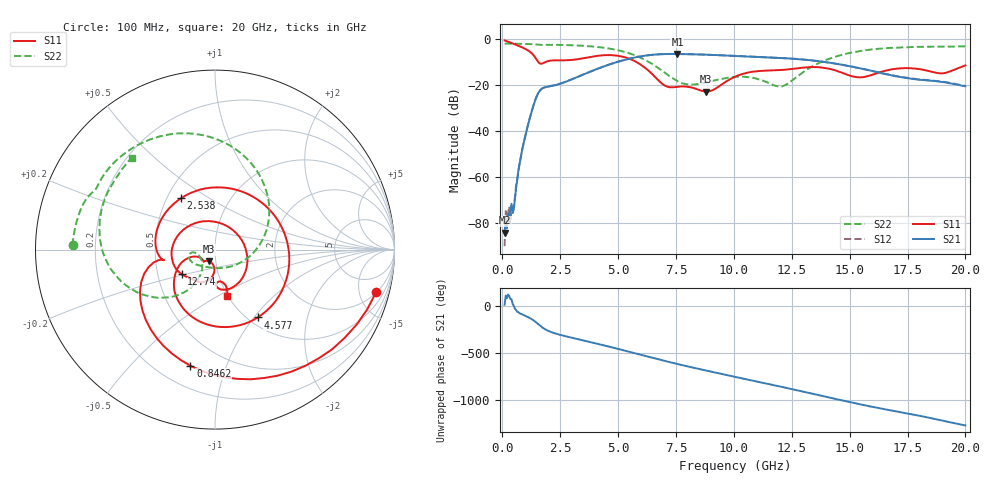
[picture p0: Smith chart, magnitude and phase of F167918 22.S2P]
!  2-Port S-parameters saved by WinCal
! VAR MeasName=S-Parameters (CALIBRATED_DATA) read from VNA (N5242A)
! VAR MeasDate=2016-11-22 10:25:49
! VAR NAME=F167918 22
! VAR FILENAME=F167918 22.S2P
! VAR DATE=2016-11-22 10:25:49
! VAR PHYS_PORTS=1,2
# Hz S DB R 50
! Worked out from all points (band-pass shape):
!   401 points, 100 MHz to 20 GHz, reference 50 ohm
!   highest |S21| = -6.49 dB at 7.562 GHz (marker M1); lowest = -84.2 dB at 100 MHz (marker M2)
!   |S21| within 3 dB of the highest: 5.137 GHz to 13.52 GHz (8.382 GHz wide, 89.9 % of centre)
!   lowest |S11| = -22.8 dB at 8.806 GHz (marker M3), VSWR 1.16, Z = 46.5 - j6.02 ohm
!   |S11| at or under -10 dB: 1.556 GHz to 1.868 GHz (311.8 MHz wide, 18.2 % of centre); 5.793 GHz to end of sweep
!   |S22| runs from -20.7 to -2.0 dB; largest |S21 - S12| = 0.005
!   S11 on the Smith chart (normalised r, x): 100 MHz: 2.07, -7.12; 846.2 MHz: 0.33, -0.76; 2.538 GHz: 0.59, +0.38; 4.577 GHz: 1.11, -1.04; 12.74 GHz: 0.66, -0.19; 20 GHz: 0.99, -0.55
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1e8  -0.64 -14.8  -84.16 17.5  -89.97 57.8  -2.00 178.3
4.4825e8  -1.91 -57.8  -75.62 26.3  -72.96 21.5  -2.05 172.6
8.4625e8  -3.59 -101.9  -48.76 -83.0  -48.78 -82.8  -2.11 166.1
1.1945e9  -5.56 -140.1  -34.13 -126.2  -34.08 -126.1  -2.21 160.2
1.54275e9  -9.85 -169.4  -23.71 171.9  -23.66 171.8  -2.48 154.7
2.53775e9  -9.29 123.3  -19.32 52.4  -19.29 52.1  -2.58 139.5
3.43325e9  -8.50 36.7  -15.71 -0.8  -15.72 -0.9  -2.93 121.2
3.9805e9  -7.51 -11.2  -13.46 -32.8  -13.45 -32.7  -3.34 108.1
4.5775e9  -7.00 -57.8  -11.24 -68.7  -11.21 -68.7  -4.09 91.5
5.62225e9  -9.13 -126.3  -8.27 -134.4  -8.23 -134.6  -6.70 54.9
6.7665e9  -18.21 -161.7  -6.65 151.7  -6.65 151.5  -12.81 -0.0
7.5625e9  -20.76 -134.9  -6.49 102.8  -6.51 102.7  -18.28 -53.3
8.80625e9  -22.84 -116.6  -6.83 32.3  -6.82 32.3  -18.79 -125.5
1.005e10  -16.41 -96.0  -7.33 -35.0  -7.33 -34.8  -16.49 -156.3
1.129375e10  -13.77 -120.7  -7.92 -100.7  -7.88 -100.7  -18.28 -172.9
1.204e10  -13.46 -131.6  -8.27 -140.6  -8.22 -140.8  -20.60 -147.9
1.27365e10  -12.73 -143.6  -8.70 -179.1  -8.68 -179.2  -16.32 -120.7
1.338325e10  -12.24 -162.7  -9.31 144.8  -9.30 144.8  -11.93 -122.5
1.5025e10  -15.99 97.6  -11.87 54.2  -11.89 54.3  -6.05 -151.8
1.67165e10  -13.39 -40.1  -15.54 -32.0  -15.52 -31.0  -3.89 176.3
1.9005e10  -14.92 -81.8  -18.65 -143.0  -18.50 -142.8  -3.34 143.7
2e10  -11.46 -75.9  -20.52 164.5  -20.34 164.8  -3.22 132.1
